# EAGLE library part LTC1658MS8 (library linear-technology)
DIGITAL/ANALOG CONVERTER
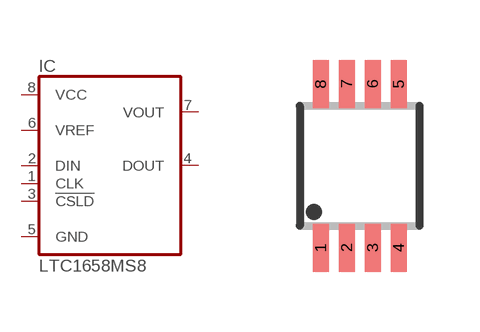
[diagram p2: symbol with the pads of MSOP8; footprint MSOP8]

Designator prefix IC

## LTC1658MS8 (OC_FARNELL: unknown; OC_NEWARK: unknown)  [MSOP8]
1  CLK  in
2  DIN  in
3  !CSLD  in
4  DOUT  out
5  GND  pwr
6  VREF  in
7  VOUT  out
8  VCC  pwr

## Footprint MSOP8 (pad centres in mm)
MSOP8
smd 0.4 x 1.2: 1 -0.975,-2.05; 2 -0.325,-2.05; 3 0.325,-2.05; 4 0.975,-2.05; 5 0.975,2.05; 6 0.325,2.05; 7 -0.325,2.05; 8 -0.975,2.05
